FUNCTION FC 76 : VOID
TITLE =BLOCK FOR OVERLOAD MEASURES
AUTHOR : Esposito
FAMILY : EGAL_srl
NAME : OVERL_M
VERSION : 0.1

BEGIN
NETWORK
TITLE =OVERLOAD TONN TRADUCER 3
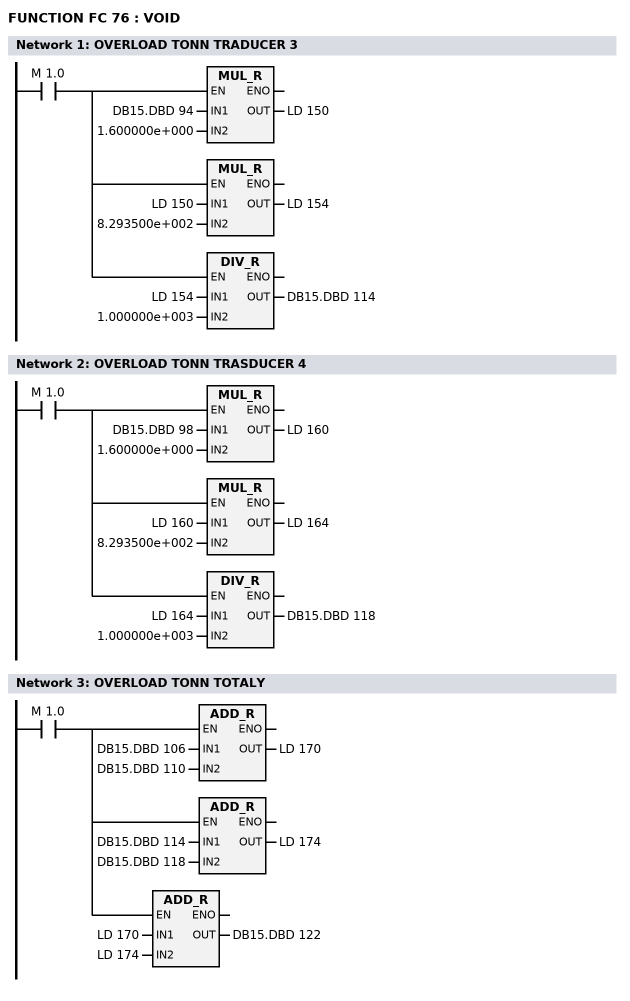
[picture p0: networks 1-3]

      U     M      1.0;
      =     L    178.0;
      U     L    178.0;
      SPBNB _001;
      L     DB15.DBD   94;
      L     1.600000e+000;
      *R    ;
      T     LD   150;
_001: NOP   0;
      U     L    178.0;
      SPBNB _002;
      L     LD   150;
      L     8.293500e+002;
      *R    ;
      T     LD   154;
_002: NOP   0;
      U     L    178.0;
      SPBNB _003;
      L     LD   154;
      L     1.000000e+003;
      /R    ;
      T     DB15.DBD  114;
_003: NOP   0;
NETWORK
TITLE =OVERLOAD TONN TRASDUCER 4

      U     M      1.0;
      =     L    178.0;
      U     L    178.0;
      SPBNB _004;
      L     DB15.DBD   98;
      L     1.600000e+000;
      *R    ;
      T     LD   160;
_004: NOP   0;
      U     L    178.0;
      SPBNB _005;
      L     LD   160;
      L     8.293500e+002;
      *R    ;
      T     LD   164;
_005: NOP   0;
      U     L    178.0;
      SPBNB _006;
      L     LD   164;
      L     1.000000e+003;
      /R    ;
      T     DB15.DBD  118;
_006: NOP   0;
NETWORK
TITLE =OVERLOAD TONN TOTALY

      U     M      1.0;
      =     L    178.0;
      U     L    178.0;
      SPBNB _007;
      L     DB15.DBD  106;
      L     DB15.DBD  110;
      +R    ;
      T     LD   170;
_007: NOP   0;
      U     L    178.0;
      SPBNB _008;
      L     DB15.DBD  114;
      L     DB15.DBD  118;
      +R    ;
      T     LD   174;
_008: NOP   0;
      U     L    178.0;
      SPBNB _009;
      L     LD   170;
      L     LD   174;
      +R    ;
      T     DB15.DBD  122;
_009: NOP   0;
END_FUNCTION

